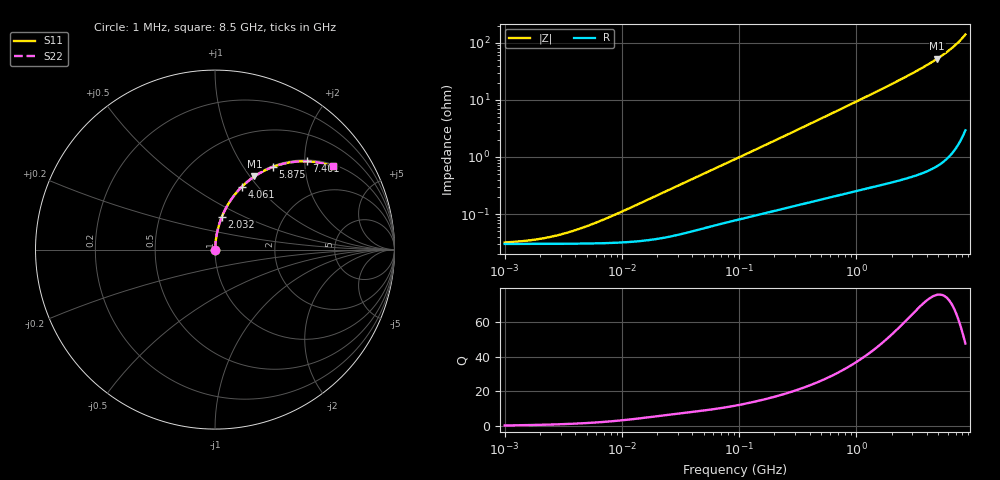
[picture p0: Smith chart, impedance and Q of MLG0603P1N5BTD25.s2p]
! S-Parameter Data Generated by TDK Corporation
! Copyright(C) 2025 TDK Corporation.
! All Rights Reserved.
! TDK P/N: MLG0603P1N5BTD25 (SMD / SMT Inductor (Coil))
! Property: L=1.5nH at 500MHz
! Size(LxWxT): 0.6x0.3x0.3mm
! Model Type: s2p (Touchstone File Format Version 1.0)
! Frequency: DC=Yes Start=1MHz Stop=8500MHz 198points Log-sweep
! Model Generated on Feb. 6, 2025
! Terms and conditions regarding TDK Simulation Models:
! 1)This simulation model is being provided solely for informational
!  purposes. Please refer to the specifications of the products in
!  terms of detailed characteristics of such products.
! 2)In no event shall TDK Corporation of any of its subsidiaries be
!  liable for any loss or damage arising, directly or indirectly,
!  from any information contained in this simulation model, including,
!  but not limited to loss or damages arising from any inaccuracies,
!  omissions or errors in connection with such information.
! 3)Any and all copyrights on this simulation model are owned by
!  TDK Corporation.  Duplication or redistribution of this simulation
!  model without prior written permission from TDK Corporation
!  is prohibited.
! 4)This simulation model is subject to any modification or change
!  without any prior notice.
! 5)Neither TDK Corporation nor any of its subsidiaries shall make any
!  warranty, express or implied, including but not limited to the
!  correctness, implied warranties of merchantability and fitness for
!  a particular purpose with respect to this simulation models.
! 6)The use of this simulation model shall be deemed to have consented
!  to the terms and conditions hereof.
! Port Assignments:
!  1 ---@@@--- 2
! Applicable Conditions:
!  Temperature = 25 degC
!  DC Bias Current = 0 A
!  Small Signal Operation
# Hz S MA R 50
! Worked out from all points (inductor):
!   197 points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, 1 MHz to 8.5 GHz, reference 50 ohm
!   read as one part in series: L = 1.68 nH near 9.169 MHz
!   highest Q = 75.9 at 4.885 GHz (marker M1), where L = 1.71 nH
!   S11 on the Smith chart (normalised r, x): 1 MHz: 1.00, +0.00; 2.032 GHz: 1.01, +0.38; 4.061 GHz: 1.01, +0.83; 5.875 GHz: 1.02, +1.37; 7.401 GHz: 1.03, +2.04; 8.5 GHz: 1.06, +2.80
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1000000  0.0003183 19.5  0.9997 -0.0  0.9997 -0.0  0.0003183 19.5
1515069  0.0003406 28.1  0.9997 -0.0  0.9997 -0.0  0.0003406 28.1
2191881  0.0003802 37.7  0.9997 -0.0  0.9997 -0.0  0.0003802 37.7
3171038  0.0004519 48.1  0.9997 -0.0  0.9997 -0.0  0.0004519 48.1
4587603  0.0005735 58.0  0.9997 -0.0  0.9997 -0.0  0.0005735 58.0
8360083  0.0009385 70.5  0.9997 -0.1  0.9997 -0.1  0.0009385 70.5
2.10461e7  0.002236 80.3  0.9996 -0.1  0.9996 -0.1  0.002236 80.3
9.219544e7  0.009132 84.6  0.9992 -0.5  0.9992 -0.5  0.009132 84.6
4.229561e8  0.03991 85.3  0.9976 -2.3  0.9976 -2.3  0.03991 85.3
9.708683e8  0.09034 83.2  0.9934 -5.2  0.9934 -5.2  0.09034 83.2
1.404574e9  0.1303 81.2  0.9885 -7.5  0.9885 -7.5  0.1303 81.2
1.940355e9  0.1799 78.5  0.9802 -10.4  0.9802 -10.4  0.1799 78.5
2.032026e9  0.1884 78.1  0.9786 -10.9  0.9786 -10.9  0.1884 78.1
2.939772e9  0.2737 73.2  0.9576 -15.9  0.9576 -15.9  0.2737 73.2
3.535948e9  0.3307 69.9  0.939 -19.3  0.939 -19.3  0.3307 69.9
4.061159e9  0.3816 66.8  0.9191 -22.4  0.9191 -22.4  0.3816 66.8
4.884749e9  0.4626 61.7  0.8805 -27.6  0.8805 -27.6  0.4626 61.7
5.87536e9  0.561 55.1  0.8203 -34.1  0.8203 -34.1  0.561 55.1
6.748056e9  0.6469 48.9  0.7532 -40.3  0.7532 -40.3  0.6469 48.9
7.400733e9  0.7091 43.9  0.6937 -45.2  0.6937 -45.2  0.7091 43.9
8.116539e9  0.7736 38.3  0.6193 -50.7  0.6193 -50.7  0.7736 38.3
8.5e9  0.8058 35.1  0.5756 -53.7  0.5756 -53.7  0.8058 35.1
